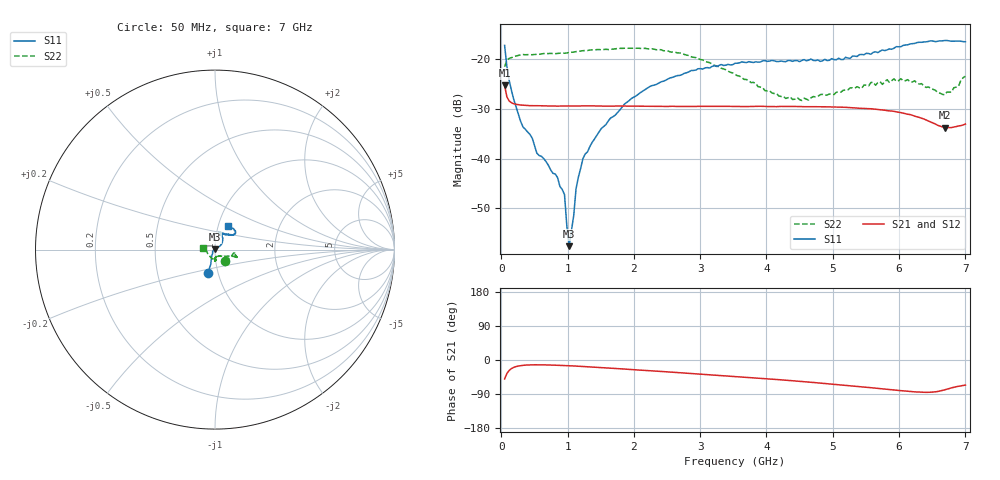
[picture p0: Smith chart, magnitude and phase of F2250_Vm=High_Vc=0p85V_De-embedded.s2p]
! Integrated Device Technology
! Corporate Headquarters
! 6024 Silver Creek Valley Road
! San Jose, CA 95138  USA
! Phone:  1-408-284-8200
! Toll Free:  1-800-223-1366
! Webpage:  http://www.idt.com/
! Timing and RF Division
! 515 Groton Road, Suite 102
! Westford, MA 01886-6024
! Device:  F2250
! Description: Voltage Variable RF Attenuator
! Frequency:  50.0 -  6000.00 MHz
! Package:  3x3 mm Thin QFN Plastic Package: 16 pin
! Ports:  2 RF, 3 DC
!  Pin  1  = GND
!  Pin  2  = NC
!  Pin  3  = RF1  = Port 1
!  Pin  4  = NC
!  Pin  5  = GND
!  Pin  6  = GND
!  Pin  7  = GND
!  Pin  8  = GND
!  Pin  9  = NC
!  Pin 10  = RF2  = Port 2
!  Pin 11  = NC
!  Pin 12  = GND
!  Pin 13  = GND
!  Pin 14  = VCNTRL
!  Pin 15  = VDD
!  Pin 16  = VMODE
! Vcntrl:  0.850 Volts
! Vmode:  +3.300 Volts
! Vdd:  +3.30  Volts
! Current:  1.309 mA
! Data:  The device was measured on a the F2250 evaluation board which has
!  individual transmission lines to the RF pins.  Data was collected
!  using a calibrated network analyzer.  The evaluation board was
!  de-embedded using a TRL calibration technique.
!  The reference plane is the edge of the package pin.
! Misc:  SN 10
!  Action Tracker AT0258
! Date Measured:  2014-11-26
! Date:  2015-10-15  MJV
! Note:
!  Integrated Device Technology supplies this data as a sample of measured
!  data at the package pin for this product.  Your particular data for this
!  product may vary.
!  Data was taken at 25 degrees C.
!  Integrated Device Technology reserves the right to change this data at anytime.
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# GHz S dB R 50
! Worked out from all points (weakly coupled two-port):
!   201 points, 50 MHz to 7 GHz, reference 50 ohm
!   highest |S21| = -25.25 dB at 50 MHz (marker M1); lowest = -33.8 dB at 6.687 GHz (marker M2)
!   lowest |S11| = -57.7 dB at 1.023 GHz (marker M3), VSWR 1.00, Z = 49.9 + j0.12 ohm
!   |S11| at or under -10 dB: start of sweep to end of sweep
!   |S22| runs from -28.3 to -17.7 dB; largest |S21 - S12| = 0.00013
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0.05  -17.16 -107.4  -25.25 -50.0  -25.23 -49.9  -21.48 -50.0
0.1195  -24.24 -110.1  -28.38 -27.4  -28.37 -27.4  -19.78 -14.4
0.29325  -32.55 -123.3  -29.19 -14.8  -29.20 -14.8  -19.06 -9.2
0.467  -35.89 -141.5  -29.32 -12.8  -29.30 -12.7  -19.04 -8.2
0.5365  -38.91 -148.9  -29.33 -12.7  -29.33 -12.7  -18.95 -9.2
0.84925  -43.86 171.8  -29.42 -13.9  -29.40 -14.0  -18.78 -13.2
0.9535  -47.26 174.8  -29.38 -14.7  -29.39 -14.7  -18.74 -14.3
0.98825  -53.53 169.4  -29.40 -14.9  -29.40 -14.9  -18.68 -14.6
1.023  -57.68 113.3  -29.40 -15.2  -29.39 -15.2  -18.57 -14.6
1.0925  -51.49 50.3  -29.40 -15.7  -29.40 -15.7  -18.52 -15.1
1.12725  -46.12 40.0  -29.40 -16.1  -29.39 -16.1  -18.41 -15.7
1.2315  -40.01 31.3  -29.40 -17.0  -29.40 -17.1  -18.22 -17.1
1.5095  -33.93 35.8  -29.41 -20.1  -29.41 -20.1  -18.04 -18.0
1.857  -29.02 36.5  -29.40 -23.9  -29.39 -23.9  -17.73 -19.4
2.37825  -24.74 44.9  -29.46 -29.8  -29.45 -29.9  -17.98 -19.9
3.525  -20.76 70.9  -29.48 -43.5  -29.48 -43.5  -22.98 -32.2
4.2895  -20.44 75.2  -29.48 -53.3  -29.48 -53.3  -27.86 -62.0
4.7065  -20.19 71.5  -29.52 -59.3  -29.51 -59.3  -27.48 -80.4
5.85325  -17.86 40.1  -30.37 -77.9  -30.36 -78.0  -24.60 -86.2
6.2355  -16.75 38.6  -31.44 -84.1  -31.42 -84.2  -24.31 -94.3
6.68725  -16.17 47.4  -33.75 -78.9  -33.76 -78.9  -27.12 -148.4
7  -16.42 62.0  -33.02 -66.1  -33.04 -66.1  -23.39 170.2
